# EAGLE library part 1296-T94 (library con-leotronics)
1.27mm SINGLE ROW FEMALE SOCKET Source: http://www.leotronics.co.uk/Conexcon/Data%20Sheets/sec.%20A/1296ing.pdf
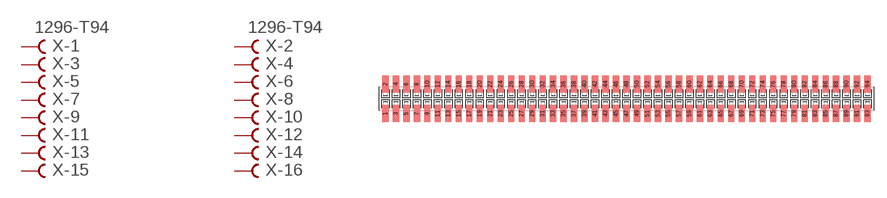
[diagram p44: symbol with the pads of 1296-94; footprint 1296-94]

Designator prefix X; gates -1=FVAL -2=FVAL -3=F -4=F -5=F -6=F -7=F -8=F -9=F -10=F -11=F -12=F -13=F -14=F -15=F -16=F -17=F -18=F -19=F -20=F -21=F -22=F -23=F -24=F -25=F -26=F -27=F -28=F -29=F -30=F -31=F -32=F -33=F -34=F -35=F -36=F -37=F -38=F -39=F -40=F -41=F -42=F -43=F -44=F -45=F -46=F -47=F -48=F -49=F -50=F -51=F -52=F -53=F -54=F -55=F -56=F -57=F -58=F -59=F -60=F -61=F -62=F -63=F -64=F -65=F -66=F -67=F -68=F -69=F -70=F -71=F -72=F -73=F -74=F -75=F -76=F -77=F -78=F -79=F -80=F -81=F -82=F -83=F -84=F -85=F -86=F -87=F -88=F -89=F -90=F -91=F -92=F -93=F -94=F

## 1296-T94 (OC_FARNELL: unknown; OC_NEWARK: unknown)  [1296-94]
1  -1:B  pas
2  -2:B  pas
3  -3:B  pas
4  -4:B  pas
5  -5:B  pas
6  -6:B  pas
7  -7:B  pas
8  -8:B  pas
9  -9:B  pas
10  -10:B  pas
11  -11:B  pas
12  -12:B  pas
13  -13:B  pas
14  -14:B  pas
15  -15:B  pas
16  -16:B  pas
17  -17:B  pas
18  -18:B  pas
19  -19:B  pas
20  -20:B  pas
21  -21:B  pas
22  -22:B  pas
23  -23:B  pas
24  -24:B  pas
25  -25:B  pas
26  -26:B  pas
27  -27:B  pas
28  -28:B  pas
29  -29:B  pas
30  -30:B  pas
31  -31:B  pas
32  -32:B  pas
33  -33:B  pas
34  -34:B  pas
35  -35:B  pas
36  -36:B  pas
37  -37:B  pas
38  -38:B  pas
39  -39:B  pas
40  -40:B  pas
41  -41:B  pas
42  -42:B  pas
43  -43:B  pas
44  -44:B  pas
45  -45:B  pas
46  -46:B  pas
47  -47:B  pas
48  -48:B  pas
49  -49:B  pas
50  -50:B  pas
51  -51:B  pas
52  -52:B  pas
53  -53:B  pas
54  -54:B  pas
55  -55:B  pas
56  -56:B  pas
57  -57:B  pas
58  -58:B  pas
59  -59:B  pas
60  -60:B  pas
61  -61:B  pas
62  -62:B  pas
63  -63:B  pas
64  -64:B  pas
65  -65:B  pas
66  -66:B  pas
67  -67:B  pas
68  -68:B  pas
69  -69:B  pas
70  -70:B  pas
71  -71:B  pas
72  -72:B  pas
73  -73:B  pas
74  -74:B  pas
75  -75:B  pas
76  -76:B  pas
77  -77:B  pas
78  -78:B  pas
79  -79:B  pas
80  -80:B  pas
81  -81:B  pas
82  -82:B  pas
83  -83:B  pas
84  -84:B  pas
85  -85:B  pas
86  -86:B  pas
87  -87:B  pas
88  -88:B  pas
89  -89:B  pas
90  -90:B  pas
91  -91:B  pas
92  -92:B  pas
93  -93:B  pas
94  -94:B  pas

## Footprint 1296-94 (pad centres in mm)
1.27mm SINGLE ROW FEMALE SOCKET Source: http://www.leotronics.co.uk/Conexcon/Data%20Sheets/sec.%20A/1296ing.pdf
smd 0.76 x 2.05: 1 -29.21,-1.78; 2 -29.21,1.78; 3 -27.94,-1.78; 4 -27.94,1.78; 5 -26.67,-1.78; 6 -26.67,1.78; 7 -25.4,-1.78; 8 -25.4,1.78; 9 -24.13,-1.78; 10 -24.13,1.78; 11 -22.86,-1.78; 12 -22.86,1.78; 13 -21.59,-1.78; 14 -21.59,1.78; 15 -20.32,-1.78; 16 -20.32,1.78; 17 -19.05,-1.78; 18 -19.05,1.78; 19 -17.78,-1.78; 20 -17.78,1.78; 21 -16.51,-1.78; 22 -16.51,1.78; 23 -15.24,-1.78; 24 -15.24,1.78; 25 -13.97,-1.78; 26 -13.97,1.78; 27 -12.7,-1.78; 28 -12.7,1.78; 29 -11.43,-1.78; 30 -11.43,1.78; 31 -10.16,-1.78; 32 -10.16,1.78; 33 -8.89,-1.78; 34 -8.89,1.78; 35 -7.62,-1.78; 36 -7.62,1.78; 37 -6.35,-1.78; 38 -6.35,1.78; 39 -5.08,-1.78; 40 -5.08,1.78; 41 -3.81,-1.78; 42 -3.81,1.78; 43 -2.54,-1.78; 44 -2.54,1.78; 45 -1.27,-1.78; 46 -1.27,1.78; 47 0,-1.78; 48 0,1.78; 49 1.27,-1.78; 50 1.27,1.78; 51 2.54,-1.78; 52 2.54,1.78; 53 3.81,-1.78; 54 3.81,1.78; 55 5.08,-1.78; 56 5.08,1.78; 57 6.35,-1.78; 58 6.35,1.78; 59 7.62,-1.78; 60 7.62,1.78; 61 8.89,-1.78; 62 8.89,1.78; 63 10.16,-1.78; 64 10.16,1.78; 65 11.43,-1.78; 66 11.43,1.78; 67 12.7,-1.78; 68 12.7,1.78; 69 13.97,-1.78; 70 13.97,1.78; 71 15.24,-1.78; 72 15.24,1.78; 73 16.51,-1.78; 74 16.51,1.78; 75 17.78,-1.78; 76 17.78,1.78; 77 19.05,-1.78; 78 19.05,1.78; 79 20.32,-1.78; 80 20.32,1.78; 81 21.59,-1.78; 82 21.59,1.78; 83 22.86,-1.78; 84 22.86,1.78; 85 24.13,-1.78; 86 24.13,1.78; 87 25.4,-1.78; 88 25.4,1.78; 89 26.67,-1.78; 90 26.67,1.78; 91 27.94,-1.78; 92 27.94,1.78; 93 29.21,-1.78; 94 29.21,1.78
